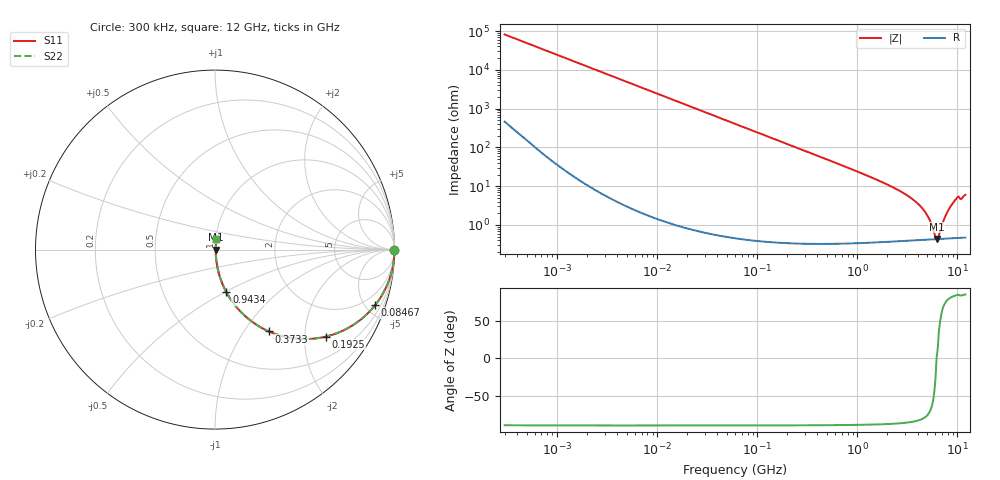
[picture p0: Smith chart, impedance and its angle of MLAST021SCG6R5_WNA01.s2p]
! MLAST021SCG6R5_WNA01  S-PARAMETER MODEL  ( General Type )
! Model Generated by TAIYO YUDEN Corporation (http://www.ty-top.com)
! Version 1.0
! TAIYO YUDEN Control No. 220901
! Copyright(c) 2022 TAIYO YUDEN CO.,LTD. All Rights Reserved.
! Product Description (link to TY-COMPAS)
! https://ds.yuden.co.jp/TYCOMPAS/or/detail?pn=MLAST021SCG6R5CWNA01&u=M
! Products Name : Multilayer Ceramic Capacitors
! Characteristics :
!  Capacitance : 6.5 pF , Rated Voltage : 25V , TCC : CG / C0G
!  Case Size : 0.25 x 0.125 / 0.0098 x 0.0049 [mm/inch] , Thickness : 0.125 / 0.0049 [mm/inch]
!  (Conditions: Temperature = 25 degC , DC Bias Current/Voltage = 0A / 0V)
! External Node Assignments :
!  1  o---| |---o  2
! GND o---------o GND
! Frequency Range : 0.3MHz  -  12000MHz  [ 401 STEP ]
# MHz S RI R 50
! Freq[MHz].  S11 Real  S11 Imag  S21 Real  S21 Imag  S12 Real  S12 Imag  S22 Real  S22 Imag
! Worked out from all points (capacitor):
!   401 points, 300 kHz to 12 GHz, reference 50 ohm
!   read as one part in series: C = 6.5 pF near 316.3 kHz
!   lowest |Z| = 432 mohm at 6.188 GHz (marker M1)
!   series resonance near 6.19 GHz, so ESL is about 100 pH
!   S11 on the Smith chart (normalised r, x): 300 kHz: open; 84.67 MHz: 1.01, -5.78; 192.5 MHz: 1.01, -2.54; 373.3 MHz: 1.01, -1.31; 943.4 MHz: 1.01, -0.51; 12 GHz: 1.01, +0.12
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0.3  1 -0.00123  8.47e-06 0.00123  8.47e-06 0.00123  1 -0.00123
1.769972  0.9999 -0.00723  5.9e-05 0.00723  5.9e-05 0.00723  0.9999 -0.00723
10.44266  0.9982 -0.0426  0.00184 0.0426  0.00184 0.0426  0.9982 -0.0426
27.10171  0.9878 -0.1093  0.0122 0.1093  0.0122 0.1093  0.9878 -0.1093
60  0.9431 -0.2311  0.0569 0.2311  0.0569 0.2311  0.9431 -0.2311
84.66778  0.8928 -0.3086  0.1072 0.3086  0.1072 0.3086  0.8928 -0.3086
192.4766  0.6173 -0.4847  0.3827 0.4847  0.3827 0.4847  0.6173 -0.4847
353.9943  0.323 -0.4653  0.677 0.4653  0.677 0.4653  0.323 -0.4653
373.2558  0.3002 -0.4559  0.6998 0.4559  0.6998 0.4559  0.3002 -0.4559
585.5907  0.1485 -0.3517  0.8515 0.3517  0.8515 0.3517  0.1485 -0.3517
943.3804  0.0632 -0.2367  0.9368 0.2367  0.9368 0.2367  0.0632 -0.2367
2088.533  0.0142 -0.1021  0.9858 0.1021  0.9858 0.1021  0.0142 -0.1021
3190.978  0.00704 -0.0558  0.993 0.0558  0.993 0.0558  0.00704 -0.0558
4270.516  0.00498 -0.0299  0.995 0.0299  0.995 0.0299  0.00498 -0.0299
5140.631  0.00441 -0.0148  0.9956 0.0148  0.9956 0.0148  0.00441 -0.0148
5868.704  0.00429 -0.00432  0.9957 0.00432  0.9957 0.00432  0.00429 -0.00432
6188.031  0.0043 -1.02e-05  0.9957 1.02e-05  0.9957 1.02e-05  0.0043 -1.02e-05
6524.734  0.00435 0.00313  0.9957 -0.00313  0.9957 -0.00313  0.00435 0.00313
7648.807  0.00473 0.0171  0.9953 -0.0171  0.9953 -0.0171  0.00473 0.0171
8966.534  0.00582 0.0357  0.9942 -0.0357  0.9942 -0.0357  0.00582 0.0357
9708.23  0.00671 0.046  0.9933 -0.046  0.9933 -0.046  0.00671 0.046
12000  0.00823 0.059  0.9918 -0.059  0.9918 -0.059  0.00823 0.059
